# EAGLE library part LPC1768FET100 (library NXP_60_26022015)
32-bit ARM Cortex-M3 microcontroller; up to 512 kB flash and 64 kB SRAM with Ethernet, USB 2.0 Host/Device/OTG, CAN The LPC1769/68/67/66/65/64/63 are ARM Cortex-M3 based microcontrollers for embedded applications featuring a high level of integration and low power consumption. The ARM Cortex-M3 is a next generation core that offers system enhancements such as enhanced debug features and a higher level of support block integration. The LPC1768/67/66/65/64/63 operate at CPU frequencies of up to 100 MHz. The LPC1769 operates at CPU frequencies of up to 120 MHz. The ARM Cortex-M3 CPU incorporates a 3-stage pipeline and uses a Harvard architecture with separate local instruction and data buses as well as a third bus for peripherals. The ARM Cortex-M3 CPU also includes an internal prefetch unit that supports speculative branching. The peripheral complement of the LPC1769/68/67/66/65/64/63 includes up to 512 kB of flash memory, up to 64 kB of data memory, Ethernet MAC, USB Device/Host/OTG interface, 8-channel general purpose DMA controller, 4 UARTs, 2 CAN channels, 2 SSP controllers, SPI interface, 3 I 2 C-bus interfaces, 2-input plus 2-output I 2 S-bus interface, 8-channel 12-bit ADC, 10-bit DAC, motor control PWM, Quadrature Encoder interface, four general purpose timers, 6-output general purpose PWM, ultra-low power Real-Time Clock (RTC) with separate battery supply, and up to 70 general purpose I/O pins. The LPC1769/68/67/66/65/64/63 are pin-compatible to the 100-pin LPC236x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
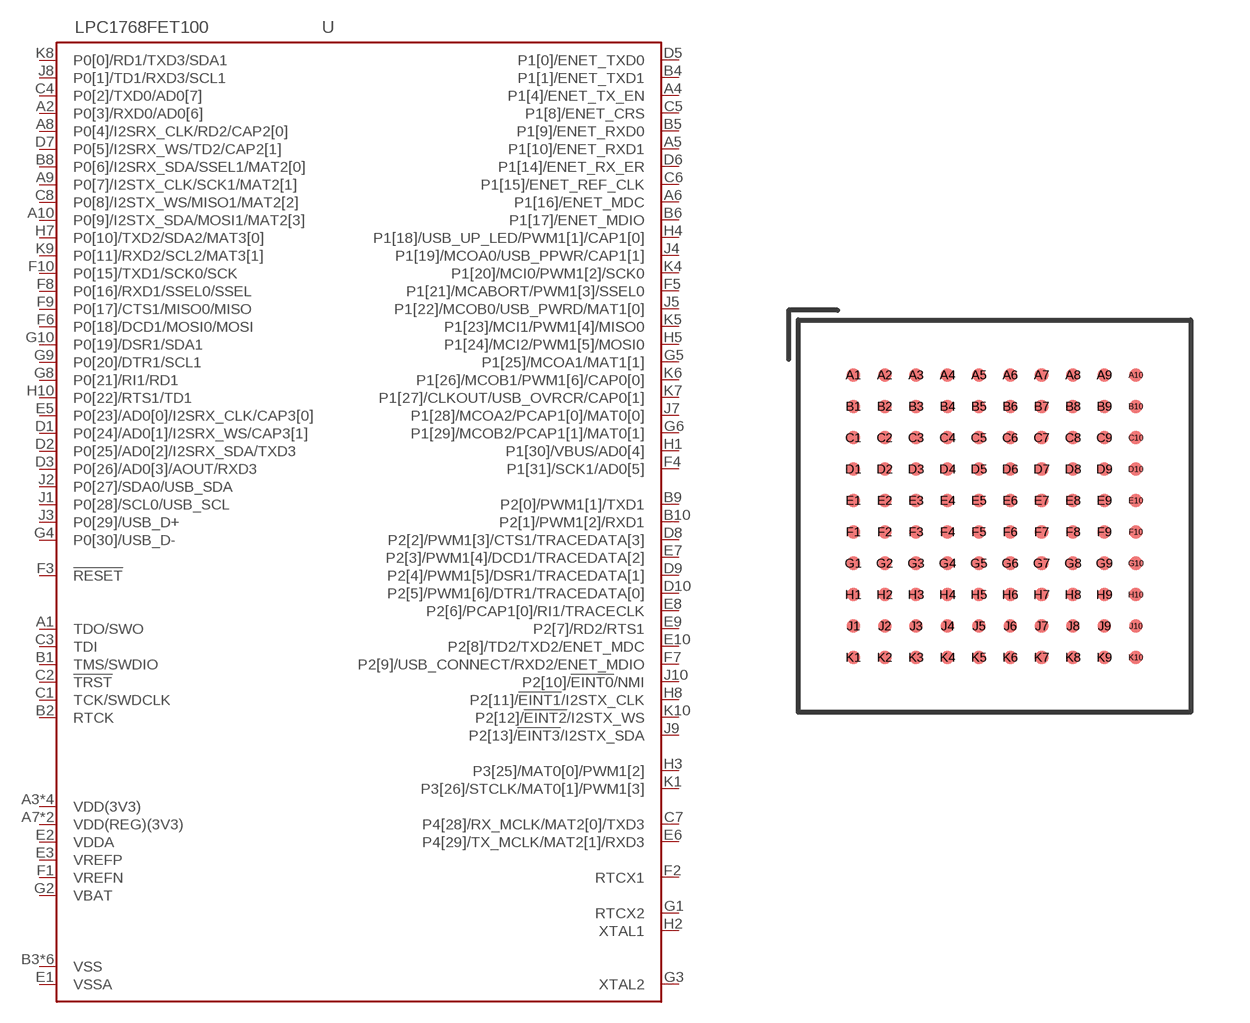
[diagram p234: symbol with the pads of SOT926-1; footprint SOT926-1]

Designator prefix U

## LPC1768FET100 (CAN: yes; DAC: yes; ETH: yes; FLASH: 512kB; I2S: yes; MHZ: 100; SRAM: 32kB; SRAM0: 16kB; SRAM1: 16kB; USB: D/H/OTG)  [SOT926-1]
A1  TDO/SWO
A2  P0[3]/RXD0/AD0[6]
A3  VDD(3V3)
A4  P1[4]/ENET_TX_EN
A5  P1[10]/ENET_RXD1
A6  P1[16]/ENET_MDC
A7  VDD(REG)(3V3)
A8  P0[4]/I2SRX_CLK/RD2/CAP2[0]
A9  P0[7]/I2STX_CLK/SCK1/MAT2[1]
A10  P0[9]/I2STX_SDA/MOSI1/MAT2[3]
B1  TMS/SWDIO
B2  RTCK
B3  VSS
B4  P1[1]/ENET_TXD1
B5  P1[9]/ENET_RXD0
B6  P1[17]/ENET_MDIO
B7  VSS
B8  P0[6]/I2SRX_SDA/SSEL1/MAT2[0]
B9  P2[0]/PWM1[1]/TXD1
B10  P2[1]/PWM1[2]/RXD1
C1  TCK/SWDCLK
C2  !TRST!
C3  TDI
C4  P0[2]/TXD0/AD0[7]
C5  P1[8]/ENET_CRS
C6  P1[15]/ENET_REF_CLK
C7  P4[28]/RX_MCLK/MAT2[0]/TXD3
C8  P0[8]/I2STX_WS/MISO1/MAT2[2]
C9  VSS
C10  VDD(3V3)
D1  P0[24]/AD0[1]/I2SRX_WS/CAP3[1]
D2  P0[25]/AD0[2]/I2SRX_SDA/TXD3
D3  P0[26]/AD0[3]/AOUT/RXD3
D5  P1[0]/ENET_TXD0
D6  P1[14]/ENET_RX_ER
D7  P0[5]/I2SRX_WS/TD2/CAP2[1]
D8  P2[2]/PWM1[3]/CTS1/TRACEDATA[3]
D9  P2[4]/PWM1[5]/DSR1/TRACEDATA[1]
D10  P2[5]/PWM1[6]/DTR1/TRACEDATA[0]
E1  VSSA
E2  VDDA
E3  VREFP
E5  P0[23]/AD0[0]/I2SRX_CLK/CAP3[0]
E6  P4[29]/TX_MCLK/MAT2[1]/RXD3
E7  P2[3]/PWM1[4]/DCD1/TRACEDATA[2]
E8  P2[6]/PCAP1[0]/RI1/TRACECLK
E9  P2[7]/RD2/RTS1
E10  P2[8]/TD2/TXD2/ENET_MDC
F1  VREFN
F2  RTCX1
F3  !RESET!
F4  P1[31]/SCK1/AD0[5]
F5  P1[21]/MCABORT/PWM1[3]/SSEL0
F6  P0[18]/DCD1/MOSI0/MOSI
F7  P2[9]/USB_CONNECT/RXD2/ENET_MDIO
F8  P0[16]/RXD1/SSEL0/SSEL
F9  P0[17]/CTS1/MISO0/MISO
F10  P0[15]/TXD1/SCK0/SCK
G1  RTCX2
G2  VBAT
G3  XTAL2
G4  P0[30]/USB_D-
G5  P1[25]/MCOA1/MAT1[1]
G6  P1[29]/MCOB2/PCAP1[1]/MAT0[1]
G7  VSS
G8  P0[21]/RI1/RD1
G9  P0[20]/DTR1/SCL1
G10  P0[19]/DSR1/SDA1
H1  P1[30]/VBUS/AD0[4]
H2  XTAL1
H3  P3[25]/MAT0[0]/PWM1[2]
H4  P1[18]/USB_UP_LED/PWM1[1]/CAP1[0]
H5  P1[24]/MCI2/PWM1[5]/MOSI0
H6  VDD(REG)(3V3)
H7  P0[10]/TXD2/SDA2/MAT3[0]
H8  P2[11]/!EINT1!/I2STX_CLK
H9  VDD(3V3)
H10  P0[22]/RTS1/TD1
J1  P0[28]/SCL0/USB_SCL
J2  P0[27]/SDA0/USB_SDA
J3  P0[29]/USB_D+
J4  P1[19]/MCOA0/USB_PPWR/CAP1[1]
J5  P1[22]/MCOB0/USB_PWRD/MAT1[0]
J6  VSS
J7  P1[28]/MCOA2/PCAP1[0]/MAT0[0]
J8  P0[1]/TD1/RXD3/SCL1
J9  P2[13]/!EINT3!/I2STX_SDA
J10  P2[10]/!EINT0!/NMI
K1  P3[26]/STCLK/MAT0[1]/PWM1[3]
K2  VDD(3V3)
K3  VSS
K4  P1[20]/MCI0/PWM1[2]/SCK0
K5  P1[23]/MCI1/PWM1[4]/MISO0
K6  P1[26]/MCOB1/PWM1[6]/CAP0[0]
K7  P1[27]/CLKOUT/USB_OVRCR/CAP0[1]
K8  P0[0]/RD1/TXD3/SDA1
K9  P0[11]/RXD2/SCL2/MAT3[1]
K10  P2[12]/!EINT2!/I2STX_WS

## Footprint SOT926-1 (pad centres in mm)
SOT926-1 TFBGA100: plastic thin fine-pitch ball grid array package; 100 balls; body 9 x 9 x 0.7 mm JEDEC: -- IEC: --
smd 0.35 x 0.35: A1 -3.6,3.6; A2 -2.8,3.6; A3 -2,3.6; A4 -1.2,3.6; A5 -0.4,3.6; A6 0.4,3.6; A7 1.2,3.6; A8 2,3.6; A9 2.8,3.6; A10 3.6,3.6; B1 -3.6,2.8; B2 -2.8,2.8; B3 -2,2.8; B4 -1.2,2.8; B5 -0.4,2.8; B6 0.4,2.8; B7 1.2,2.8; B8 2,2.8; B9 2.8,2.8; B10 3.6,2.8; C1 -3.6,2; C2 -2.8,2; C3 -2,2; C4 -1.2,2; C5 -0.4,2; C6 0.4,2; C7 1.2,2; C8 2,2; C9 2.8,2; C10 3.6,2; D1 -3.6,1.2; D2 -2.8,1.2; D3 -2,1.2; D4 -1.2,1.2; D5 -0.4,1.2; D6 0.4,1.2; D7 1.2,1.2; D8 2,1.2; D9 2.8,1.2; D10 3.6,1.2; E1 -3.6,0.4; E2 -2.8,0.4; E3 -2,0.4; E4 -1.2,0.4; E5 -0.4,0.4; E6 0.4,0.4; E7 1.2,0.4; E8 2,0.4; E9 2.8,0.4; E10 3.6,0.4; F1 -3.6,-0.4; F2 -2.8,-0.4; F3 -2,-0.4; F4 -1.2,-0.4; F5 -0.4,-0.4; F6 0.4,-0.4; F7 1.2,-0.4; F8 2,-0.4; F9 2.8,-0.4; F10 3.6,-0.4; G1 -3.6,-1.2; G2 -2.8,-1.2; G3 -2,-1.2; G4 -1.2,-1.2; G5 -0.4,-1.2; G6 0.4,-1.2; G7 1.2,-1.2; G8 2,-1.2; G9 2.8,-1.2; G10 3.6,-1.2; H1 -3.6,-2; H2 -2.8,-2; H3 -2,-2; H4 -1.2,-2; H5 -0.4,-2; H6 0.4,-2; H7 1.2,-2; H8 2,-2; H9 2.8,-2; H10 3.6,-2; J1 -3.6,-2.8; J2 -2.8,-2.8; J3 -2,-2.8; J4 -1.2,-2.8; J5 -0.4,-2.8; J6 0.4,-2.8; J7 1.2,-2.8; J8 2,-2.8; J9 2.8,-2.8; J10 3.6,-2.8; K1 -3.6,-3.6; K2 -2.8,-3.6; K3 -2,-3.6; K4 -1.2,-3.6; K5 -0.4,-3.6; K6 0.4,-3.6; K7 1.2,-3.6; K8 2,-3.6; K9 2.8,-3.6; K10 3.6,-3.6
